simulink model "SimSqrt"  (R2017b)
settings: Solver=VariableStepAuto  StartTime=0.0  StopTime=10.0  RelTol=1e-3

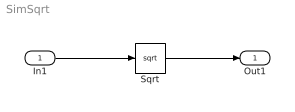
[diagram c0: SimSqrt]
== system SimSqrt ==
  In1 : Inport
  Sqrt : Sqrt
  Out1 : Outport
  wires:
  In1/1 -> Sqrt/1
  Sqrt/1 -> Out1/1
